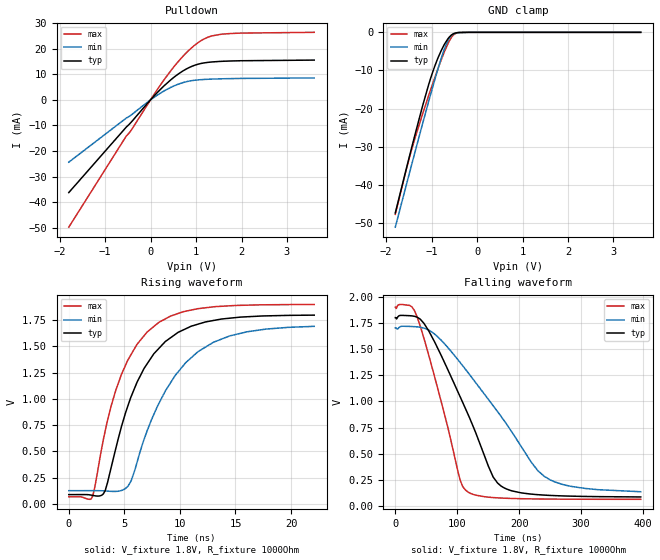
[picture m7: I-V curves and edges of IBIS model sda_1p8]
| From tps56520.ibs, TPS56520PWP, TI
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|   sda_1p8 Model
[Model]   sda_1p8
Model_type   I/O_open_drain
Polarity   Non-Inverting
Vinl = 0.6
Vinh = 1.26
Vmeas = 0.9
Vref = 1.8
Cref = 2pF
Rref = 1000
|   typ   min   max
|   (nom PVT)   (fast PVT)   (slow PVT)
C_comp   4.277e-13   3.594e-13   5.102e-13
| Where nom  PVT is Nominal Process, 1.8V, 27C
|   Fast PVT is Strong Process,  1.9V, -40C
|   Slow PVT is Weak Process,   1.7V, 125C
[Voltage Range]   1.8   1.7   1.9
|Junction Temperature
[Temperature Range]   27   125   -40
[Pullup Reference]   1.8   1.7   1.9
[Pulldown Reference]   0   0   0
[Power Clamp Reference]   1.8   1.7   1.9
[GND Clamp Reference]   0   0   0
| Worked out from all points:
|   slope of the pulldown table from 0 to 0.27 V, typ, clamps not added: 53.9 ohm
|   GND clamp passes 1 mA (typ) near -0.59 V on its own axis
|   falling waveform, V_fixture 1.8V, R_fixture 1000Ohm: 20-80 % time 74.6ns typ, 114ns min, 47.7ns max; typ from 1.8 V to 0.09 V
|   rising waveform, V_fixture 1.8V, R_fixture 1000Ohm: 20-80 % time 3.88ns typ, 4.61ns min, 3.44ns max; typ from 0.088 V to 1.8 V
[Pulldown]
|   Voltage   I(typ)   I(min)   I(max)
-1.8V     -36.23mA   -24.35mA   -49.76mA
-532.8mV  -10.59mA   -7.073mA   -14.08mA
-397.8mV  -8.136mA   -5.516mA   -11.07mA
163.5mV   3.166mA    2.048mA    4.468mA
584.5mV   9.796mA    5.975mA    14.48mA
792mV     12.13mA    7.126mA    18.52mA
966.4mV   13.52mA    7.671mA    21.33mA
1.113V    14.25mA    7.911mA    23.18mA
1.255V    14.65mA    8.055mA    24.46mA
1.544V    15.05mA    8.233mA    25.64mA
1.981V    15.3mA     8.38mA     26.11mA
3.6V      15.56mA    8.583mA    26.41mA
[GND Clamp]
|   Voltage   I(typ)   I(min)   I(max)
-1.8V     -47.37mA   -51.1mA    -47.74mA
-1.562V   -36.01mA   -40.25mA   -36.14mA
-1.438V   -30.17mA   -34.63mA   -30.66mA
-1.19V    -18.89mA   -23.53mA   -21.08mA
-1.021V   -11.97mA   -16.18mA   -14.99mA
-874.8mV  -7.111mA   -10.12mA   -9.986mA
-729mV    -3.361mA   -4.691mA   -5.379mA
-642.6mV  -1.696mA   -2.189mA   -3.014mA
-553.6mV  -606.9uA   -707.9uA   -1.154mA
-505.8mV  -297.8uA   -357.4uA   -532.5uA
-411.1mV  -51.26uA   -85.02uA   -60.41uA
3.6V      0A         0A         0A
[POWER Clamp]
|   Voltage   I(typ)   I(min)   I(max)
-1.8V     0A         0A         0A
0V        0A         0A         0A
3.6V      0A         0A         0A
[Ramp]
R_load = 1000
|   typ   min   max
dV/dt_r   1.02745/3.89324e-09   0.944921/4.68108e-09   1.09998/3.44789e-09
dV/dt_f   1.02713/7.46648e-08   0.942152/1.14349e-07   1.09995/4.76939e-08
[Falling Waveform]
V_fixture = 1.8V
V_fixture_min = 1.7V
V_fixture_max = 1.9V
R_fixture = 1000Ohm
|   Time   V(typ)   V(min)   V(max)
0s        1.8V       1.7V       1.9V
23.23ns   1.818V     1.716V     1.916V
35.47ns   1.803V     1.711V     1.804V
53.74ns   1.676V     1.681V     1.447V
104.9ns   1.043V     1.371V     247.3mV
113.8ns   926.1mV    1.304V     153.5mV
158ns     280.2mV    959.8mV    83.78mV
177.4ns   171.3mV    803.1mV    77.44mV
250ns     104.2mV    252.8mV    69.37mV
396.4ns   89.6mV     139.4mV    66.94mV
[Rising Waveform]
V_fixture = 1.8V
V_fixture_min = 1.7V
V_fixture_max = 1.9V
R_fixture = 1000Ohm
|   Time   V(typ)   V(min)   V(max)
0s        87.58mV    125.1mV    66.71mV
2.034ns   82.44mV    125.4mV    49.23mV
3.103ns   93.67mV    123.7mV    607.8mV
4.23ns    527.7mV    118mV      1.083V
5.334ns   938.3mV    169.4mV    1.373V
6.778ns   1.291V     615mV      1.602V
8.108ns   1.481V     956.8mV    1.729V
10.54ns   1.669V     1.347V     1.836V
13.02ns   1.747V     1.54V      1.877V
22.09ns   1.798V     1.691V     1.899V
